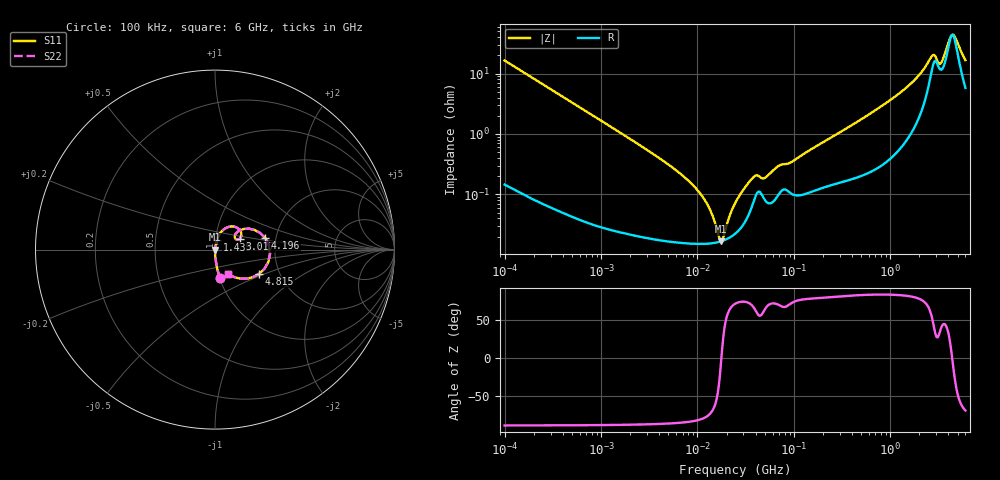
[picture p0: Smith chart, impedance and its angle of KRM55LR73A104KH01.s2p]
!Murata Part Number: KRM55LR73A104KH01
!These Parameters are Measured in Series Mode Connection
!Data Generated on Jan 08, 2026
!  o--ll--o
!Port1  Port2
!  o------o
!Operation Temp=25[degC], DC Bias Voltage=0[V]
!Freq. Start=100[kHz] Stop=6[GHz] 401[Steps]
# Hz S RI R 50
!Freq.(Hz) S11(Real) S11(Imag) S21(Real) S21(Imag) S12(Real) S12(Imag) S22(Real) S22(Imag)
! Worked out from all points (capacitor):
!   401 points, 100 kHz to 6 GHz, reference 50 ohm
!   read as one part in series: C = 96.7 nF near 105.7 kHz
!   lowest |Z| = 16.7 mohm at 17.61 MHz (marker M1)
!   series resonance near 17.7 MHz, so ESL is about 840 pH
!   S11 on the Smith chart (normalised r, x): 100 kHz: 1.00, -0.33; 1.435 GHz: 1.01, +0.11; 3.017 GHz: 1.31, +0.16; 4.196 GHz: 1.76, +0.24; 4.815 GHz: 1.57, -0.46; 6 GHz: 1.12, -0.31
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100000  0.0277 -0.1596  0.9723 0.1596  0.9723 0.1596  0.0277 -0.1596
631452  0.00105 -0.0262  0.9989 0.0262  0.9989 0.0262  0.00105 -0.0262
3987316  0.00019 -0.00401  0.9998 0.00401  0.9998 0.00401  0.00019 -0.00401
7302625  0.000159 -0.00193  0.9998 0.00193  0.9998 0.00193  0.000159 -0.00193
1.073283e7  0.000152 -0.00101  0.9998 0.00101  0.9998 0.00101  0.000152 -0.00101
1.337449e7  0.000154 -0.000553  0.9998 0.000553  0.9998 0.000553  0.000154 -0.000553
1.760885e7  0.000167 -1e-05  0.9998 1e-05  0.9998 1e-05  0.000167 -1e-05
1.860466e7  0.000172 9.91e-05  0.9998 -9.91e-05  0.9998 -9.91e-05  0.000172 9.91e-05
2.517799e7  0.000231 0.000733  0.9998 -0.000733  0.9998 -0.000733  0.000231 0.000733
3.909733e7  0.000845 0.00181  0.9992 -0.00181  0.9992 -0.00181  0.000845 0.00181
5.007898e7  0.000803 0.00169  0.9992 -0.00169  0.9992 -0.00169  0.000803 0.00169
6.966265e7  0.001 0.00279  0.999 -0.00279  0.999 -0.00279  0.001 0.00279
1.546735e8  0.00114 0.00559  0.9989 -0.00559  0.9989 -0.00559  0.00114 0.00559
9.76689e8  0.00497 0.035  0.995 -0.035  0.995 -0.035  0.00497 0.035
1.435462e9  0.0104 0.0553  0.9896 -0.0553  0.9896 -0.0553  0.0104 0.0553
2.628996e9  0.1042 0.1286  0.8958 -0.1286  0.8958 -0.1286  0.1042 0.1286
3.016594e9  0.1376 0.0602  0.8624 -0.0602  0.8624 -0.0602  0.1376 0.0602
3.367428e9  0.1103 0.0778  0.8897 -0.0778  0.8897 -0.0778  0.1103 0.0778
3.863894e9  0.1901 0.1165  0.8099 -0.1165  0.8099 -0.1165  0.1901 0.1165
4.19625e9  0.2807 0.0633  0.7193 -0.0633  0.7193 -0.0633  0.2807 0.0633
4.814911e9  0.2456 -0.1351  0.7544 0.1351  0.7544 0.1351  0.2456 -0.1351
6e9  0.0751 -0.137  0.9249 0.137  0.9249 0.137  0.0751 -0.137
